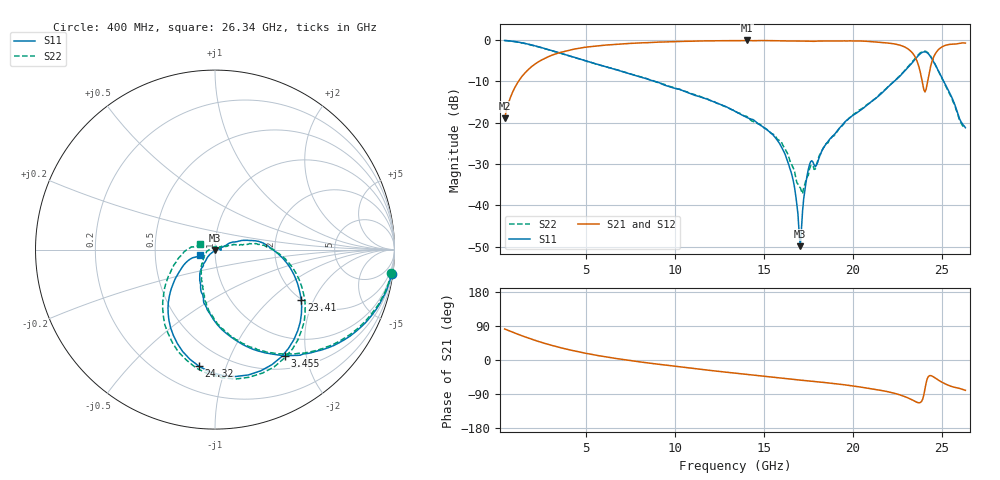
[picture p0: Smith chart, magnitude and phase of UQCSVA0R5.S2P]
!  Part Number  UQCSVA0R5  Mounting Orientation: Horizontal
!  Description: Ultra Low ESR Microwave capacitors
!  Application: Coupling, Bypass, Tuning, DC Block
!  Filters, Matching
# GHZ S DB R 50
! Freq  |S11|  S11 Ph  |S21|  S21 Ph  |S12|  S12 Ph  |S22|  S22 Ph
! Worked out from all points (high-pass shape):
!   400 points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, 400 MHz to 26.34 GHz, reference 50 ohm
!   highest |S21| = -0.07 dB at 14.05 GHz (marker M1); lowest = -18.9 dB at 400 MHz (marker M2)
!   |S21| within 3 dB of the highest: 3.455 GHz to 23.35 GHz (19.9 GHz wide, 148 % of centre); 24.68 GHz to end of sweep
!   lowest |S11| = -49.9 dB at 17.04 GHz (marker M3), VSWR 1.01, Z = 50.2 - j0.27 ohm
!   |S11| at or under -10 dB: 8.857 GHz to 22.33 GHz (13.47 GHz wide, 86.4 % of centre); 25.12 GHz to end of sweep
!   |S22| runs from -37.2 to -0.1 dB; largest |S21 - S12| = 0.0073
!   S11 on the Smith chart (normalised r, x): 400 MHz: 1, -14; 3.455 GHz: 0.69, -1.63; 23.41 GHz: 1.98, -1.61; 24.32 GHz: 0.35, -0.81; 26.34 GHz: 0.85, -0.05
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0.4  -0.06 -7.9  -18.93 81.9  -18.93 81.8  -0.08 -7.7
1.44  -0.68 -27.2  -8.45 62.8  -8.47 62.8  -0.71 -26.5
3.455  -3.01 -56.7  -3.07 33.6  -3.08 33.5  -3.05 -55.6
4.755  -4.71 -70.5  -1.83 19.7  -1.83 19.8  -4.74 -69.8
9.045  -10.21 -100.9  -0.46 -11.2  -0.45 -11.2  -10.25 -98.9
13.4  -17.28 -125.1  -0.11 -35.0  -0.10 -35.1  -17.28 -123.7
14.05  -18.76 -125.8  -0.07 -38.1  -0.06 -38.3  -18.53 -130.1
16.195  -27.72 -137.5  -0.18 -49.1  -0.17 -49.3  -26.42 -167.1
16.715  -35.58 -131.3  -0.19 -51.5  -0.18 -51.8  -31.65 170.2
17.04  -49.92 -57.6  -0.21 -53.1  -0.19 -53.2  -35.72 127.9
17.235  -38.40 12.2  -0.21 -54.0  -0.19 -54.2  -35.69 83.5
17.69  -29.22 -2.9  -0.28 -56.1  -0.26 -56.4  -30.26 24.1
17.885  -30.70 0.4  -0.25 -56.6  -0.23 -56.8  -31.25 19.6
19.575  -19.70 23.4  -0.18 -65.7  -0.16 -66.0  -19.68 15.5
22.045  -11.08 6.4  -0.72 -84.5  -0.70 -84.8  -11.11 4.5
23.41  -5.10 -30.2  -3.40 -107.0  -3.40 -107.3  -4.89 -28.6
23.8  -3.27 -53.4  -7.82 -112.2  -7.80 -112.5  -3.06 -52.3
24.06  -2.82 -75.1  -12.53 -76.4  -12.51 -76.7  -2.66 -75.0
24.32  -3.66 -97.8  -7.40 -41.3  -7.39 -41.6  -3.50 -99.0
24.645  -6.00 -119.5  -3.27 -47.8  -3.26 -48.2  -5.96 -123.7
25.165  -10.39 -140.6  -1.32 -62.2  -1.31 -62.7  -10.52 -150.5
26.335  -21.21 -160.1  -0.70 -80.0  -0.69 -80.5  -21.10 159.4
